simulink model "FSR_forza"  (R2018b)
settings: Solver=FixedStepDiscrete  StartTime=0.0  StopTime=inf  RelTol=1e-3  EnableMultiTasking=on
libraries: arduinolib x2, dsparch4 x1

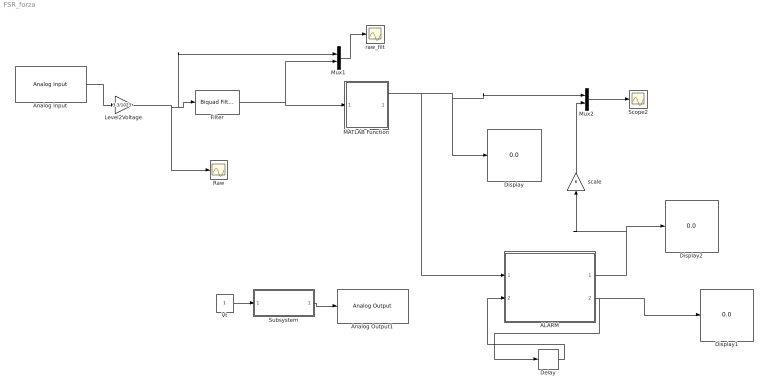
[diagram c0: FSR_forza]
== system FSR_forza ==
  ALARM : MATLAB Function  TreatAsAtomicUnit=on
  Analog Input : arduinolib/Analog Input  pinNumber=0  ReadResultsOnly=off  ConversionTriggerSource=Software  ExternalTriggerType=uint32(0)  OutputDataType=uint16  EnableConversionCompleteNotify=off  EnableOuputStatus=off  SampleTime=0.01  blockPlatform=arduino
  Analog Output1 : arduinolib/Analog Output  DACpin=DAC0  blockPlatform=arduino
  Delay : Delay  DelayLength=1  InitialCondition=0
  Display : Display
  Display1 : Display
  Display2 : Display
  Filter : dsparch4/Biquad Filter  Tag=BlockMethodSubSystem  FilterSource=Dialog parameters  CoeffSource=Specify via dialog  FilterObject=BQF  IIRFiltStruct=Direct form II  BiQuadCoeffs=[1 2 1 1 -1.17564273339370851 0.590215815099901175;1 2 1 1 -0.911519710238840486 0.232953700834604677]  ScaleValues=[0.10364327042654814;0.0803584976489410407;1]  IC=0  ICnum=0  ICden=0  a0Flag=Warning  optimizeScaleValues=on  ScaleValueMode=Specify via input port (g)  InputProcessing=Columns as channels (frame based)  roundingMode=Floor  overflowMode=off  scaleValueFracLength=14  denProdOutputFracLength=30  denAccumFracLength=30  secondMemoryFracLength=15
  "Level2Voltage " : Gain  Gain=3.3/1023  OutDataTypeStr=double
  MATLAB Function : MATLAB Function  TreatAsAtomicUnit=on
  Mux1 : Mux  Inputs=2
  Mux2 : Mux  Inputs=2
  Raw : Scope
  Scope2 : Scope
  Subsystem : Subsystem
  Vt : Constant  SampleTime=0.01
  raw_filt : Scope
  scale : Gain  Gain=6  OutDataTypeStr=double
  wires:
  MATLAB Function/1(F) -> ALARM/1(in1), Mux2/1, Display/1
  "Level2Voltage "/1 -> Mux1/1, Filter/1, Raw/1
  Mux1/1 -> raw_filt/1
  Analog Input/1 -> "Level2Voltage "/1
  ALARM/2(counter) -> Display1/1, Delay/1
  Delay/1 -> ALARM/2(in2)
  ALARM/1(alarm) -> Display2/1, scale/1
  Mux2/1 -> Scope2/1
  scale/1 -> Mux2/2
  Filter/1 -> Mux1/2, MATLAB Function/1(y)
  Subsystem/1(Out1) -> Analog Output1/1
  Vt/1 -> Subsystem/1(In1)

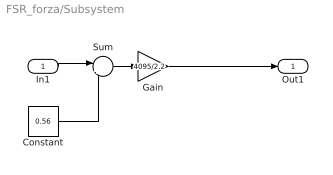
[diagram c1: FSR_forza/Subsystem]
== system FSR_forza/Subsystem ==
  In1 : Inport
  Constant : Constant  Value=0.56
  Gain : Gain  Gain=4095/2.2  OutDataTypeStr=uint16
  Sum : Sum  Inputs=|+-
  Out1 : Outport
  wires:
  In1/1 -> Sum/1
  Constant/1 -> Sum/2
  Sum/1 -> Gain/1
  Gain/1 -> Out1/1

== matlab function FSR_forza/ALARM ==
function [alarm,counter]  = allarme(in1,in2)

alarm=0;

if (in1 < 6 )
    counter=0;
else
    counter=in2+1;
end
    
if (counter>200) && (in1 > 6) 
    alarm=1;
end

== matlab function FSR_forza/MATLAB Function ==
function F  = conversione(y)
s=3.33e-3;
o=0.99;

W=y-o;

c=1/(s);
F=c*W;
